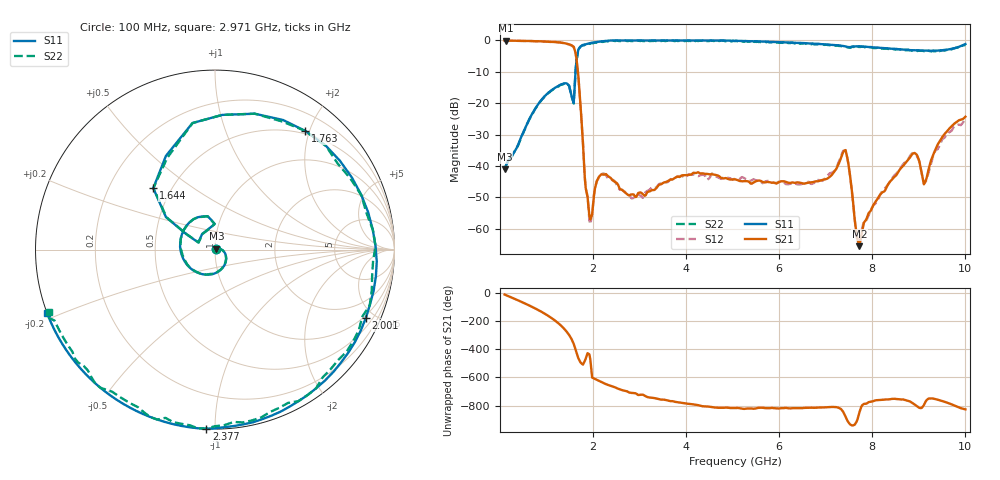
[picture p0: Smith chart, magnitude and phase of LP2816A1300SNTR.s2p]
!	AVX	THIN	FILM	OPERATION
!	LP2816S	High	Performance	Low	Pass	Filters
!	P/N	LP2816A1300SNTR
!	Created	10	January	2017
!Instrument:	"HEWLETT PACKARD,8720ES,US39172150,7.62 "
#	MHz	S	dB	R	50
!	Frq	S11(dB)	S11(deg)	S21(dB)	S21(deg)	S12(dB)	S12(deg)	S22(dB)	S22(deg)
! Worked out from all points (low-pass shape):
!   501 points, 100 MHz to 10 GHz, reference 50 ohm
!   highest |S21| = -0.06 dB at 119.8 MHz (marker M1); lowest = -65.5 dB at 7.723 GHz (marker M2)
!   |S21| within 3 dB of the highest: start of sweep to 1.606 GHz
!   lowest |S11| = -41.0 dB at 100 MHz (marker M3), VSWR 1.02, Z = 50.8 + j0.442 ohm
!   |S11| at or under -10 dB: start of sweep to 1.623 GHz
!   |S22| runs from -41.0 to 0.0 dB; largest |S21 - S12| = 0.023
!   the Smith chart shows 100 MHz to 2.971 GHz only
!   S11 on the Smith chart (normalised r, x): 100 MHz: 1.02, +0.01; 1.644 GHz: 0.40, +0.36; 1.763 GHz: 0.45, +1.94; 2.001 GHz: 0.88, -4.48; 2.377 GHz: 0.00, -0.95; 2.971 GHz: 0.00, -0.18
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100  -41.00 29.2  -0.06 -14.0  -0.04 -14.3  -41.00 29.1
119.8  -40.21 25.8  -0.06 -16.7  -0.05 -16.9  -40.41 25.6
634.6  -24.97 -17.3  -0.17 -92.2  -0.17 -92.3  -25.07 -17.4
1070.2  -16.30 -116.2  -0.42 -171.7  -0.47 -171.7  -16.50 -116.4
1406.8  -13.65 132.8  -0.93 93.7  -0.97 92.5  -13.65 132.7
1545.4  -18.00 101.6  -1.60 25.9  -1.68 24.9  -18.20 101.5
1644.4  -6.28 135.1  -5.79 -63.6  -6.00 -65.0  -6.28 135.0
1763.2  -1.61 52.7  -28.04 -144.2  -27.99 -142.8  -1.61 52.7
1901.8  -0.97 1.5  -52.94 -73.1  -53.46 -67.2  -0.97 1.3
2000.8  -0.70 -24.3  -52.35 115.4  -52.10 114.1  -0.90 -24.4
2377  -0.01 -92.8  -43.77 61.1  -44.48 64.5  -0.01 -93.0
2971  0.00 -159.4  -48.60 -5.0  -49.10 -10.6  -0.10 -159.5
3406.6  0.00 164.6  -46.15 -33.5  -45.92 -32.5  -0.10 164.5
4198.6  0.00 113.5  -42.24 -73.0  -42.93 -76.6  -0.20 113.3
5050  -0.11 69.3  -44.23 -97.7  -43.94 -89.0  -0.21 69.3
6713.2  -1.02 -7.5  -45.15 -94.7  -45.62 -93.2  -1.02 -7.7
7426  -1.91 -42.4  -34.92 -159.3  -35.13 -162.5  -2.11 -42.4
7723  -1.85 -54.4  -65.54 -127.5  -64.26 -122.7  -2.05 -54.4
8356.6  -2.56 -89.4  -45.45 -35.8  -45.53 -39.9  -2.66 -89.5
8871.4  -3.09 -122.0  -36.06 -63.1  -35.87 -73.7  -3.29 -122.2
9128.8  -3.23 -141.6  -45.25 -62.4  -45.32 -72.5  -3.33 -141.7
10000  -1.16 117.9  -24.29 -106.2  -24.82 -111.8  -1.36 117.8
